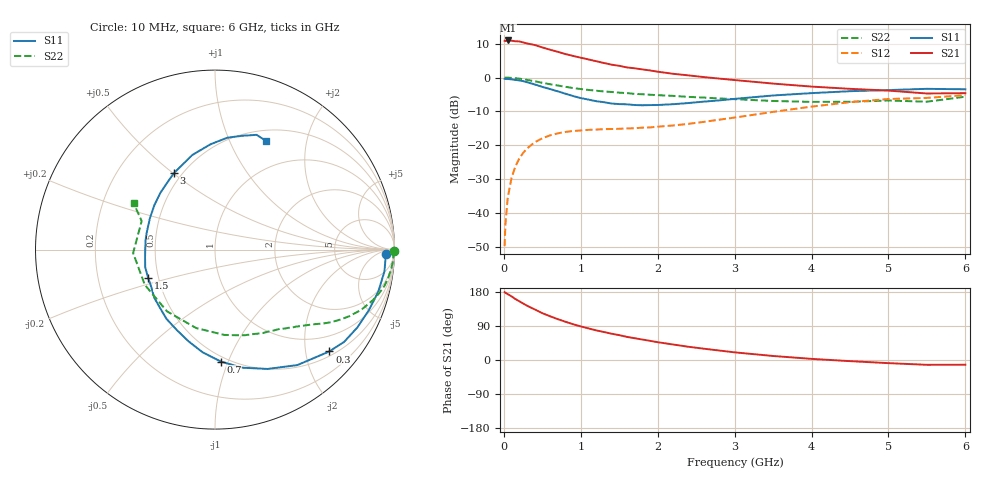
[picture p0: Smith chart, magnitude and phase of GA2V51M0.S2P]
! Infineon Technologies  Discrete & RF Semiconductors
! BF775
! Si NPN RF Bipolar Junction Transistor in SOT23
! VCE = 2.5 V  IC = 1 mA
! Common Emitter S-Parameters:  May  1996
# GHz  S  MA  R  50
!  f  S11  S21  S12  S22
! GHz  MAG  ANG  MAG  ANG  MAG  ANG  MAG  ANG
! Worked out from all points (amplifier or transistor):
!   36 points, 10 MHz to 6 GHz, reference 50 ohm
!   highest |S21| = 11.0 dB at 50 MHz (marker M1)
!   |S21| within 3 dB of that: start of sweep to 643.4 MHz
!   unconditionally stable (mu >= 1): 1.404 GHz to end of sweep
!   at 250 MHz: K = 0.21, MSG = 16.4 dB, |S12| = -22.3 dB
!   at 1.4 GHz: K = 1.00, MSG = 9.5 dB, |S12| = -15.2 dB
!   at 6 GHz: K = 1.05, MAG = -1.0 dB, |S12| = -5.2 dB
!   S11 on the Smith chart (normalised r, x): 10 MHz: 32, -18; 300 MHz: 0.60, -2.50; 700 MHz: 0.46, -0.94; 1.5 GHz: 0.44, -0.16; 3 GHz: 0.45, +0.50; 6 GHz: 0.63, +1.38
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0.01  0.9537 -1.5  3.487 179.1  0.0032 90.9  0.9991 -0.6
0.02  0.9514 -2.7  3.456 177.5  0.0066 86.1  0.9935 -1.2
0.05  0.9519 -7.3  3.532 173.9  0.0164 85.1  0.9951 -3.2
0.1  0.9394 -14.5  3.506 167.9  0.0328 80.8  0.987 -6.4
0.15  0.921 -21.6  3.436 160.9  0.0483 76.3  0.9772 -9.6
0.2  0.9039 -28.7  3.415 155.1  0.0629 72.1  0.9631 -12.5
0.3  0.8531 -41.7  3.191 143.5  0.089 64.6  0.9233 -17.8
0.4  0.7902 -54.5  3.027 133.6  0.1099 57.5  0.8811 -22.4
0.5  0.7267 -66.2  2.788 123.6  0.1262 51.6  0.835 -26.4
0.7  0.6247 -87.0  2.404 107.9  0.1491 42.9  0.7617 -32.1
0.9  0.5318 -106.1  2.086 94.4  0.1618 37.2  0.6991 -36.4
1.1  0.4714 -124.9  1.851 83.4  0.1681 33.5  0.6551 -40.2
1.2  0.4462 -133.5  1.741 78.2  0.1698 32.1  0.6375 -42.0
1.5  0.4044 -157.2  1.489 65.6  0.1743 30.9  0.5972 -46.9
1.8  0.3885 178.9  1.318 54.0  0.1812 32.8  0.5651 -51.9
2.2  0.4028 154.2  1.135 40.9  0.195 35.9  0.5348 -60.6
3  0.4832 118.4  0.917 20.2  0.2555 40.2  0.4782 -83.8
3.5  0.5421 103.5  0.813 10.6  0.31 38.5  0.4496 -103.5
4.5  0.6273 83.7  0.68 -3.0  0.4315 27.3  0.4376 -153.4
5  0.6518 76.6  0.64 -8.3  0.4806 19.5  0.4565 -177.6
5.5  0.68 70.1  0.58 -12.7  0.499 10.7  0.4386 158.7
6  0.669 64.7  0.587 -12.5  0.5481 6.0  0.5202 150.4
